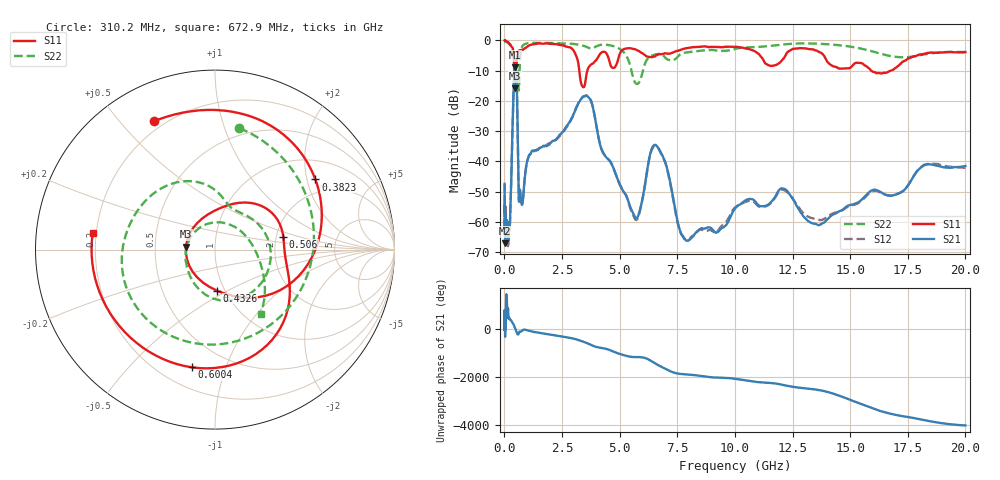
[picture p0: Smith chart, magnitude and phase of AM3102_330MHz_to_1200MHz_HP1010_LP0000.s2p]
! Date/Time: Tue, Sep 11, 2018 5:18 PM
! Network Analyzer: Agilent Technologies E8362B Rev: A.07.50.63
! Sweep from 0.010 to 20.000 GHz, 1601 Points, Sweep Type: LOG
! Power Supply: 4.949 V, 0.001 A
# Hz S DB R 50
!freq MagS11 AngS11 MagS21 AngS21 MagS12 AngS12 MagS22 AngS22
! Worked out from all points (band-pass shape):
!   1601 points, 10 MHz to 20 GHz, reference 50 ohm
!   highest |S21| = -8.88 dB at 471.2 MHz (marker M1); lowest = -67.1 dB at 38.91 MHz (marker M2)
!   |S21| within 3 dB of the highest: 423.5 MHz to 526.7 MHz (103.2 MHz wide, 21.7 % of centre)
!   lowest |S11| = -15.8 dB at 449.3 MHz (marker M3), VSWR 1.39, Z = 36.1 + j1.28 ohm
!   |S11| at or under -10 dB: 425.5 MHz to 476.4 MHz (50.82 MHz wide, 11.3 % of centre); 3.25 GHz to 3.597 GHz (347 MHz wide, 10.1 % of centre); 15.91 GHz to 16.77 GHz (850.3 MHz wide, 5.2 % of centre)
!   |S22| runs from -16.5 to -0.2 dB; largest |S21 - S12| = 0.0071
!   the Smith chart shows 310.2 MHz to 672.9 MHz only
!   S11 on the Smith chart (normalised r, x): 310.2 MHz: 0.16, +0.62; 382.3 MHz: 1.54, +2.25; 432.6 MHz: 0.92, -0.44; 506 MHz: 2.18, +0.37; 600.4 MHz: 0.33, -0.77; 672.9 MHz: 0.19, +0.07
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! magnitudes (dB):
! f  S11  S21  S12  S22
! 10 MHz  0.0  -47.8  -47.0  -0.2
! 35.55 MHz  0.0  -63.3  -64.4  -0.2
! 38.91 MHz  0.0  -67.1  -62.9  -0.2
! 48.64 MHz  -0.1  -58.0  -54.7  -0.3
! 126.4 MHz  -0.4  -64.2  -65.9  -0.6
! 238.9 MHz  -1.2  -60.6  -59.6  -1.5
! 310.2 MHz  -2.0  -42.0  -42.2  -3.2
! 382.3 MHz  -3.3  -20.7  -20.7  -5.6
! 432.6 MHz  -12.8  -10.7  -10.7  -5.7
! 447.2 MHz  -15.8  -9.5  -9.5  -6.1
! 449.3 MHz  -15.8  -9.3  -9.4  -6.2
! 471.2 MHz  -11.2  -8.9  -9.0  -6.8
! 506 MHz  -8.2  -9.6  -9.6  -10.3
! 600.4 MHz  -3.5  -43.6  -43.6  -13.0
! 672.9 MHz  -3.3  -49.3  -49.7  -7.1
! 1.59 GHz  -1.0  -35.4  -35.3  -0.8
! 3.599 GHz  -9.9  -18.5  -18.3  -2.3
! 5.652 GHz  -2.9  -58.3  -58.9  -13.7
! 6.549 GHz  -5.2  -34.5  -34.8  -4.6
! 7.958 GHz  -2.5  -66.1  -66.3  -3.9
! 13.68 GHz  -3.9  -61.0  -59.4  -1.1
! 20 GHz  -3.9  -41.5  -42.1  -3.8
